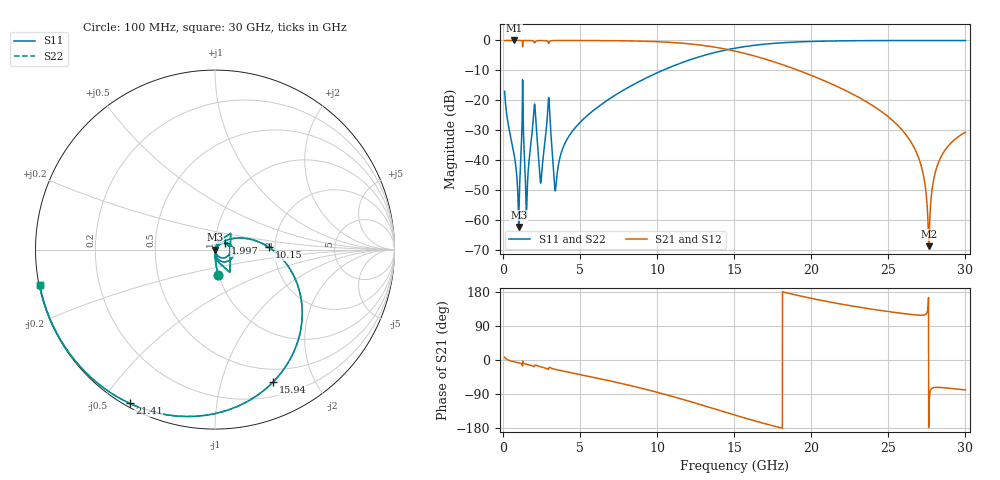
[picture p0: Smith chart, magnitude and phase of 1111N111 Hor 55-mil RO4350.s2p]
# GHz S MA R 50
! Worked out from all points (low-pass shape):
!   3201 points, 100 MHz to 30 GHz, reference 50 ohm
!   highest |S21| = -0.01 dB at 707.3 MHz (marker M1); lowest = -68.8 dB at 27.63 GHz (marker M2)
!   |S21| within 3 dB of the highest: start of sweep to 14.54 GHz
!   lowest |S11| = -62.4 dB at 1.016 GHz (marker M3), VSWR 1.00, Z = 50.1 - j0.00188 ohm
!   |S11| at or under -10 dB: start of sweep to 10.36 GHz
!   |S22| runs from -62.4 to 0.0 dB; largest |S21 - S12| = 0
!   S11 on the Smith chart (normalised r, x): 100 MHz: 1.00, -0.28; 1.997 GHz: 1.12, +0.08; 10.15 GHz: 1.85, +0.06; 15.94 GHz: 0.35, -1.47; 21.41 GHz: 0.01, -0.59; 30 GHz: 0.00, -0.10
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0.1  0.141 -82.5  0.9897 7.4  0.9897 7.4  0.141 -82.5
0.7073438  0.01279 -92.1  0.9993 -4.5  0.9993 -4.5  0.01279 -92.1
1.015688  0.0007619 -1.4  0.9991 -7.5  0.9991 -7.5  0.0007619 -1.4
1.267969  0.2199 1.4  0.7849 -12.3  0.7849 -12.3  0.2199 1.4
1.585656  0.004157 59.9  0.9985 -11.9  0.9985 -11.9  0.004157 59.9
1.996781  0.06703 31.4  0.9544 -17.5  0.9544 -17.5  0.06703 31.4
2.454625  0.004271 4.5  0.9958 -18.0  0.9958 -18.0  0.004271 4.5
2.977875  0.1034 -37.0  0.9003 -20.0  0.9003 -20.0  0.1034 -37.0
3.417031  0.003406 8.9  0.9968 -24.9  0.9968 -24.9  0.003406 8.9
3.968313  0.01799 54.5  0.9976 -29.8  0.9976 -29.8  0.01799 54.5
5.089563  0.04512 48.8  0.9968 -39.1  0.9968 -39.1  0.04512 48.8
10.06978  0.2932 3.5  0.9522 -85.9  0.9522 -85.9  0.2932 3.5
10.15387  0.2998 2.6  0.9501 -86.8  0.9501 -86.8  0.2998 2.6
15.05  0.742 -55.8  0.6635 -145.5  0.6635 -145.5  0.742 -55.8
15.93766  0.8064 -66.5  0.5838 -156.1  0.5838 -156.1  0.8064 -66.5
20.03956  0.9623 -108.0  0.2584 162.3  0.2584 162.3  0.9623 -108.0
21.41309  0.9798 -119.1  0.1826 151.3  0.1826 151.3  0.9798 -119.1
25.01978  0.9956 -143.0  0.0523 127.7  0.0523 127.7  0.9956 -143.0
26.88853  0.9969 -153.4  0.01226 118.6  0.01226 118.6  0.9969 -153.4
27.62669  0.997 -157.2  0.0003642 -156.7  0.0003642 -156.7  0.997 -157.2
28.31812  0.9969 -160.6  0.009995 -72.4  0.009995 -72.4  0.9969 -160.6
30  0.9965 -168.6  0.02922 -79.0  0.02922 -79.0  0.9965 -168.6
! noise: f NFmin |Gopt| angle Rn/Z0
0.1  0.0006817  0.7399  1.109  0.000525
3.417  0.01344  0.5936  24.81  0.005808
6.743  0.016  0.421  45.41  0.003959
10.06  0.02382  0.4424  62.5  0.005469
13.39  0.03586  0.5226  78.27  0.008437
16.7  0.05783  0.6484  95.49  0.01489
20.03  0.1071  0.7892  114.8  0.03141
23.35  0.2558  0.9058  134.3  0.09115
26.67  1.588  0.9838  152.4  1.308
30  0.9033  0.971  168.5  0.07324
